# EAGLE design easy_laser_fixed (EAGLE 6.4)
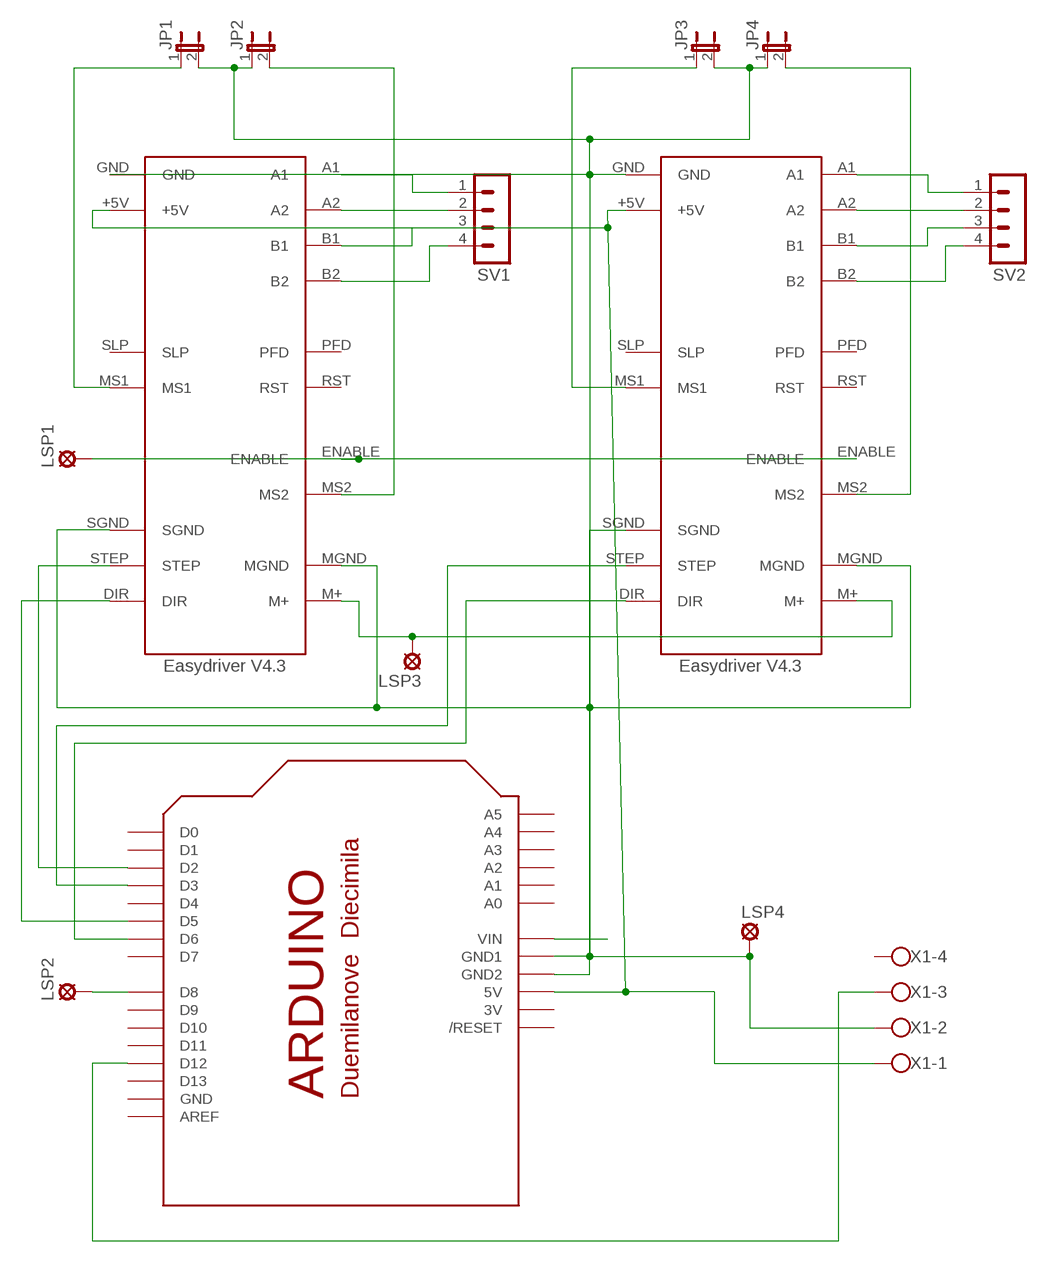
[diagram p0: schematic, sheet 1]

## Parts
JP1  JP1E  [JP1]
JP2  JP1E  [JP1]
JP3  JP1E  [JP1]
JP4  JP1E  [JP1]
LSP1  LSP11  [LSP11]
LSP2  LSP11  [LSP11]
LSP3  LSP11  [LSP11]
LSP4  LSP11  [LSP11]
SV1  MA04-1  [MA04-1]
SV2  MA04-1  [MA04-1]
U$1  EASYDRIVER  [EASYDRIVER]
U$2  EASYDRIVER  [EASYDRIVER]
U$4  ARDUINO-NOHOLE  [ARDUINO-NOHOLE]
X1  W237-4  [W237-4]

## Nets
GND: JP1.2 JP2.1 JP3.2 JP4.1 LSP4.MP U$1.GND U$1.MGND U$1.SGND U$2.GND U$2.MGND U$2.SGND U$4.GND1 U$4.GND2 X1.2
N$1: U$4.D12 X1.3
N$2: SV1.1 U$1.A1
N$3: U$2.+5V U$4.5V X1.1
N$4: JP1.1 U$1.MS1
N$5: JP2.2 U$1.MS2
N$6: JP4.2 U$2.MS2
N$7: U$1.STEP U$4.D2
N$8: U$2.STEP U$4.D3
N$9: U$1.DIR U$4.D5
N$10: U$2.DIR U$4.D6
N$11: LSP1.MP U$1.ENABLE U$2.ENABLE
N$12: JP3.1 U$2.MS1
N$13: SV1.2 U$1.A2
N$14: LSP2.MP U$4.D8
N$15: U$4.VIN
N$16: LSP3.MP U$1.M+ U$2.M+
N$17: SV1.3 U$1.B1
N$18: SV1.4 U$1.B2
N$19: SV2.1 U$2.A1
N$20: SV2.2 U$2.A2
N$21: SV2.3 U$2.B1
N$22: SV2.4 U$2.B2
N$23: U$1.+5V
Unconnected: U$1.PFD U$1.RST U$1.SLP U$2.PFD U$2.RST U$2.SLP U$4.A0 U$4.A1 U$4.A2 U$4.A3 U$4.A4 U$4.A5 U$4.AREF U$4.D0 U$4.D1 U$4.D4 U$4.D7 U$4.D9 U$4.D10 U$4.D11 U$4.D13 U$4.RESET(/RESET) X1.4

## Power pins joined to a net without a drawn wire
3V: U$4.3V
GND: U$4.GND

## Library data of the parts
JP1-JP4 = jumper:JP1E: JUMPER
LSP1-LSP4 = solpad:LSP11: SOLDER PAD
SV1 SV2 = con-lstb:MA04-1: PIN HEADER
U$1 U$2 = easydriver:EASYDRIVER: Easydriver V4.3
U$4 = adafruit:ARDUINO: Arduino Diecimila/Duemilanove Make a shield with ease, this package has all the named pins as well as the two mounting drill holes and an outline of the USB and DC power connector. The outline is on the DIMENSION layer, so if your board house uses it they will cut the outline to match.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
X1 = con-wago-500:W237-4: WAGO SCREW CLAMP; OC_FARNELL: unknown; OC_NEWARK: unknown

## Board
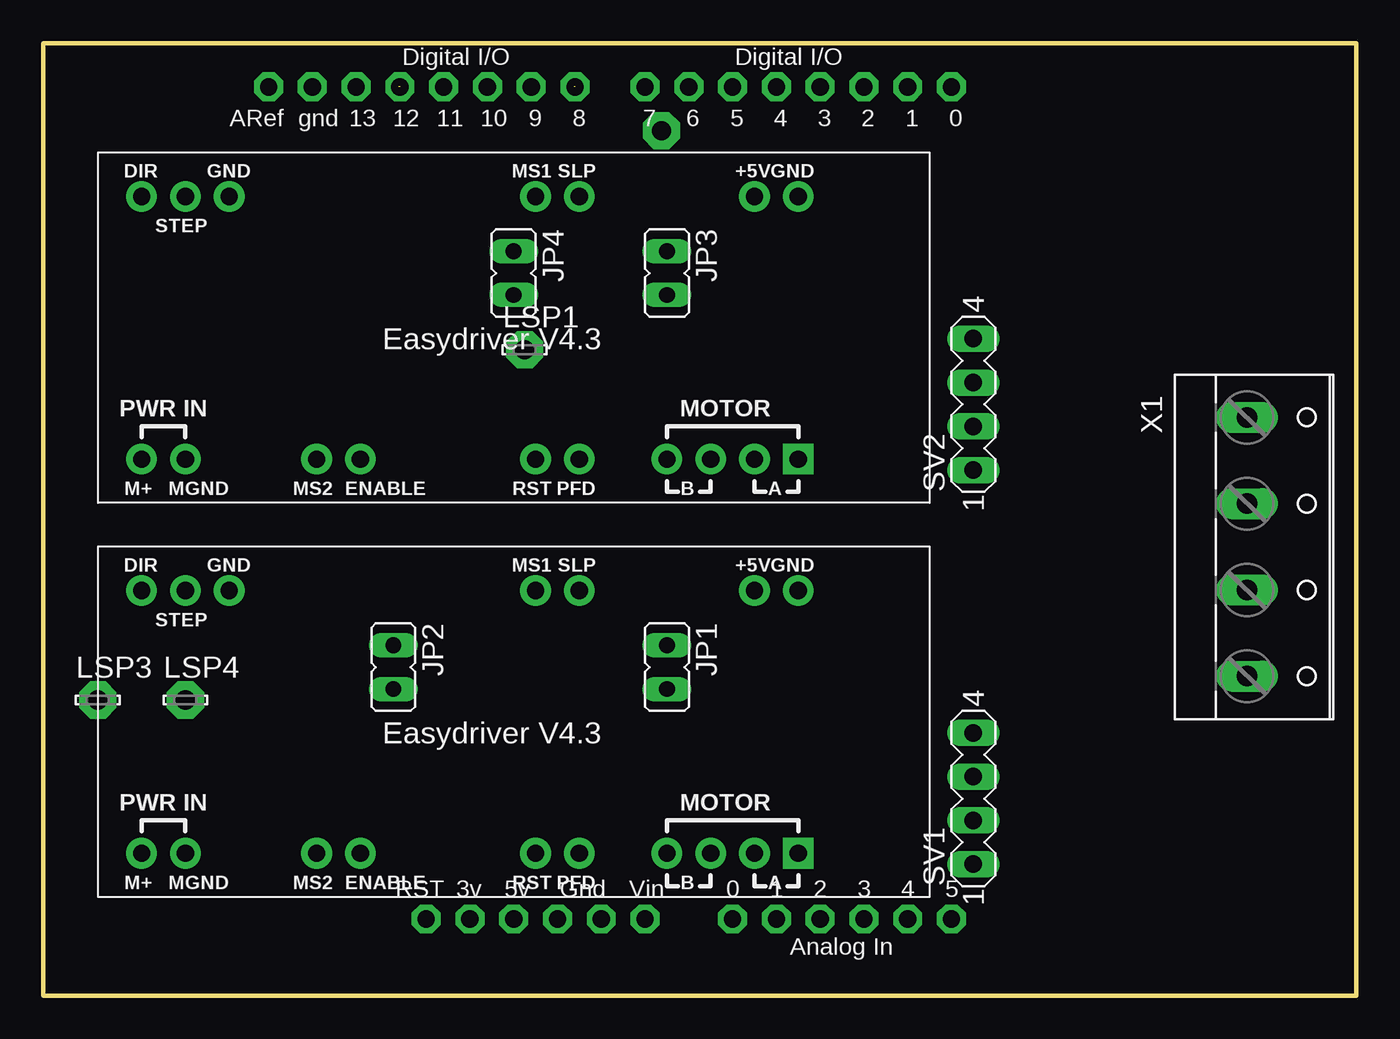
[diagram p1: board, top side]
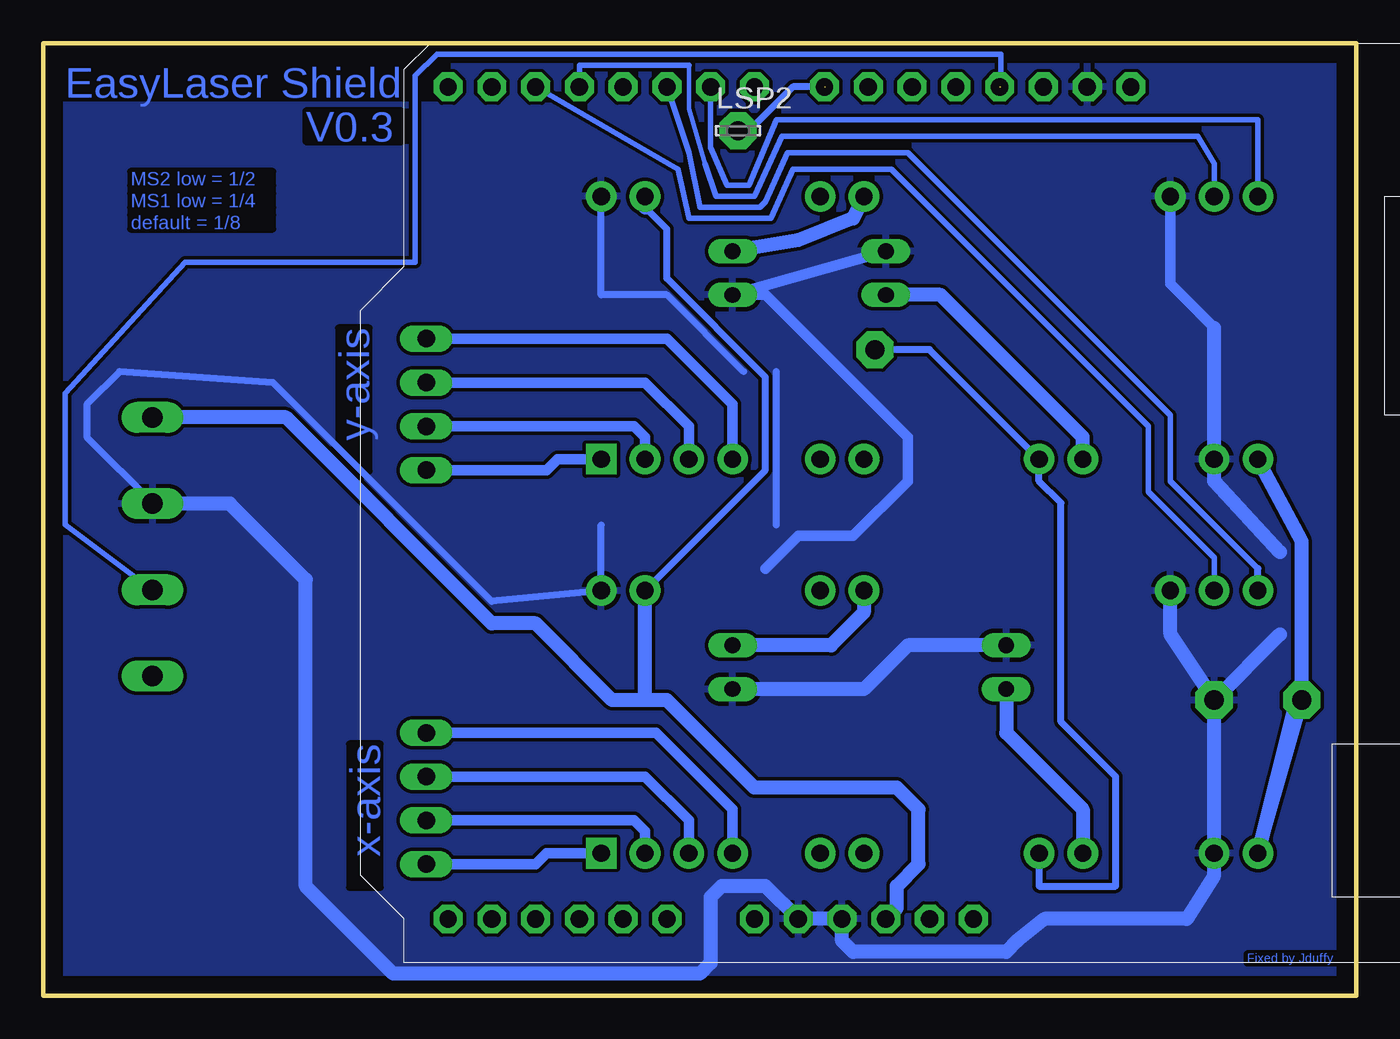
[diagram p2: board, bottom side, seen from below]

Size 76.2 x 55.25 mm. Coordinates in mm from the lower left corner, seen from the top.
Outline: 0,55.25 0,0 76.2,0 76.2,55.25 0,55.25
Copper layers (1*16): Top 0.035mm / dielectric 1.5mm / Bottom 0.035mm
Design rules "default": minimum track width 10mil, minimum drill 24mil, track to track 8mil, track to pad 8mil, pad to pad 8mil, via to via 8mil, smd to smd 8mil, copper to edge 40mil, drill to drill 8mil, minimum pad ring 10mil, minimum via ring 8mil, stop-mask expansion 4mil, vias tented up to drill 0mil, thermal gap 10mil

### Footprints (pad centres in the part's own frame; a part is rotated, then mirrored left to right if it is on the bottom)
JP1 = drill 0.914 long: 1 0,-1.27; 2 0,1.27
LSP11 = drill 1.118 pad 2.159 octagon: MP 0,0
MA04-1 = drill 1.016 long: 1 -3.81,0; 2 -1.27,0; 3 1.27,0; 4 3.81,0
EASYDRIVER = drill 1 pad 1.778: +5V -13.97,-7.62; A2 -13.97,7.62; B1 -11.43,7.62; B2 -8.89,7.62; DIR 21.59,-7.62; ENABLE 8.89,7.62; GND -16.51,-7.62; M+ 21.59,7.62; MGND 19.05,7.62; MS1 -1.27,-7.62; MS2 11.43,7.62; PFD -3.81,7.62; RST -1.27,7.62; SGND 16.51,-7.62; SLP -3.81,-7.62; STEP 19.05,-7.62 | drill 1 pad 1.778 square: A1 -16.51,7.62
ARDUINO-NOHOLE = drill 1 pad 1.676 octagon: 3V 35.56,2.54; 5V 38.1,2.54; A0 50.8,2.54; A1 53.34,2.54; A2 55.88,2.54; A3 58.42,2.54; A4 60.96,2.54; A5 63.5,2.54; AREF 23.876,50.8; D0 63.5,50.8; D1 60.96,50.8; D2 58.42,50.8; D3 55.88,50.8; D4 53.34,50.8; D5 50.8,50.8; D6 48.26,50.8; D7 45.72,50.8; D8 41.656,50.8; D9 39.116,50.8; D10 36.576,50.8; D11 34.036,50.8; D12 31.496,50.8; D13 28.956,50.8; GND 26.416,50.8; GND1 43.18,2.54; GND2 40.64,2.54; RESET 33.02,2.54; VIN 45.72,2.54
W237-4 = drill 1.194 long: 1 -7.5,-1.27; 2 -2.5,-1.27; 3 2.5,-1.27; 4 7.5,-1.27

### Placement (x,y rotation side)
JP1  36.2,19.05 180 top
JP2  20.32,19.05 180 top
JP3  36.2,41.91 180 top
JP4  27.3,41.91 180 top
LSP1  27.94,37.47 0 top
LSP2  35.88,50.16 0 bottom
LSP3  3.18,17.15 0 top
LSP4  8.26,17.15 0 top
SV1  53.97,11.43 90 top
SV2  53.97,34.29 90 top
U$1  27.3,15.87 180 top
U$2  27.3,38.73 180 top
U$4  -10.79,1.91 0 top
X1  71.12,26.03 270 top

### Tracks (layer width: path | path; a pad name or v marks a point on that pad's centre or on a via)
GND
  Bottom 0.406: 43.81,27.3 U$1.GND 50.16,22.86 62.86,35.56 71.75,36.2 73.66,34.29 73.66,32.39 69.85,28.58 | 33.66,27.3 33.66,36.2 | 35.56,36.2 40,40.64 43.81,40.64 U$2.GND
  Bottom 0.61: U$2.SGND 10.79,41.27 8.26,38.73 | JP4.1 JP3.2 34.29,40.64 26.03,32.39 26.03,29.84 29.21,26.67 32.38,26.67 34.29,24.77
  Bottom 0.813: 8.26,38.73 U$2.MGND 8.26,29.84 4.45,25.72 | LSP4.MP 4.45,20.95 | U$1.SGND 10.79,20.95 LSP4.MP | LSP4.MP U$1.MGND 8.26,6.98 9.84,4.45 18.1,4.45 19.69,3.18 20.32,2.54 29.21,2.54 29.84,3.18 U$4.GND2 U$4.GND1 34.29,6.35 36.83,6.35 37.46,5.71 37.46,1.91 38.1,1.27 55.88,1.27 60.96,6.35 60.96,24.13 65.36,28.54 X1.2 | JP2.1 26.03,20.32 28.57,17.78 JP1.2
  pour Bottom: 0.32,54.93 0.32,0.32 75.56,0.32 75.56,54.93
N$1  (1 unrouted)
  Bottom 0.305: 20.64,52.7 20.64,54.61 53.34,54.61 54.61,53.34 54.61,42.55 67.94,42.55 74.93,34.93 74.93,27.3 69.81,23.49 X1.3
N$2
  Bottom 0.61: U$1.A1 46.99,8.26 47.62,7.62 SV1.1
N$3
  Bottom 0.406: 41.27,45.72 40,44.45 40,41.59 34.29,35.88 34.29,30.48 41.27,23.49
  Bottom 0.813: U$4.5V 26.67,5.08 26.67,6.35 25.4,7.62 25.4,10.79 26.67,12.06 34.92,12.06 40,17.15 41.27,17.15 | 41.27,17.15 43.18,17.15 47.62,21.59 50.16,21.59 62.11,33.54 X1.1 | 41.27,17.15 41.27,23.49 | 41.27,45.72 U$2.+5V
N$4
  Bottom 0.813: U$1.MS1 28.57,22.23 30.48,20.32 JP1.1
N$5
  Bottom 0.813: JP2.2 20.32,15.24 15.88,10.79 U$1.MS2
N$6
  Bottom 0.813: U$2.MS2 15.88,32.39 24.13,40.64 JP4.2
N$7
  Bottom 0.305: U$4.D2 39.37,47.94 38.73,45.09 33.97,45.09 32.7,47.94 26.99,47.94 12.06,33.02 12.06,29.21 8.26,25.4 U$1.STEP
N$8
  Bottom 0.254: 37.78,48.26 38.73,51.44 38.73,53.98
  Bottom 0.305: 37.78,48.26 37.15,46.36 34.92,46.36 33.34,49.85 9.21,49.85 8.26,48.26 U$2.STEP | U$4.D3 45.09,53.98 38.73,53.98
N$9
  Bottom 0.305: U$4.D5 38.73,48.9 38.1,45.72 34.61,45.72 34.29,46.04 33.02,48.9 26.03,48.9 10.79,33.66 10.79,29.84 5.72,24.77
  Bottom 0.406: U$1.DIR 5.72,24.77
N$10
  Bottom 0.305: U$2.DIR 5.72,50.8 33.66,50.8 35.24,46.99 36.51,46.99 37.46,49.21 U$4.D6
N$11
  Bottom 0.406: U$1.ENABLE 18.41,6.35 13.97,6.35 13.97,12.7 17.15,15.87 17.15,28.58 18.41,29.84 U$2.ENABLE 24.77,37.47 LSP1.MP
N$12
  Bottom 0.813: U$2.MS1 29.21,45.09 32.38,43.82 JP3.1
N$13
  Bottom 0.61: SV1.2 41.91,10.16 41.27,9.53 U$1.A2
N$14  (1 unrouted)
  Bottom 0.406: 30.8,52.7 32.7,52.7 35.24,50.16 LSP2.MP
N$16
  Bottom 0.813: U$2.M+ 3.18,26.35 LSP3.MP | LSP3.MP 3.49,17.15 U$1.M+ LSP3.MP
N$17
  Bottom 0.61: SV1.3 41.27,12.7 38.73,10.16 U$1.B1
N$18
  Bottom 0.61: SV1.4 40.64,15.24 36.2,10.79 U$1.B2
N$19
  Bottom 0.61: SV2.1 46.99,30.48 46.35,31.12 U$2.A1
N$20
  Bottom 0.61: SV2.2 41.91,33.02 41.27,32.39 U$2.A2
N$21
  Bottom 0.61: SV2.3 41.27,35.56 38.73,33.02 U$2.B1
N$22
  Bottom 0.61: SV2.4 40,38.1 36.2,34.29 U$2.B2

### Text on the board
Bottom: EasyLaser Shield | V0.3 | MS2 low = 1/2 | MS1 low = 1/4 | default = 1/8 | y-axis | x-axis | Fixed by Jduffy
